PROGRAM AlarmsAndEventsCX7000
VAR
	events: ARRAY[0..7] OF ST_event;
	fbEvent_0: EventController;
	fbEvent_1: EventController;
	fbEvent_2: EventController;
	fbEvent_3: EventController;
	confirmAll: BOOL;
	clearAll: BOOL;
	resetAll: BOOL;
	initEvents : BOOL := FALSE;
	
END_VAR


IF NOT initEvents THEN
	initEvents := TRUE;
	
	// Info message
	events[0].severity := 0;
	events[0].needs_confirmation := FALSE;
	events[0].display_text := 'Nov izdelek na vhodnem traku.';
	events[0].cause_text := 'Prožena je fotocelica na vhodu';
	events[0].remedy_text := '';
	
	// Warning
	events[1].severity := 1;
	events[1].needs_confirmation := FALSE;
	events[1].display_text := 'Končan izdelek čaka na izhodu.';
	events[1].cause_text := 'Prožena je fotocelica na izhodu';
	events[1].remedy_text := 'Odstrani izdelek na izhodu.';
	
	// Error
	events[2].severity := 2;
	events[2].needs_confirmation := TRUE;
	events[2].display_text := 'Potiskač 1 v okvari.';
	events[2].cause_text := 'Aktivni sta obe končni stikali.';
	events[2].remedy_text := 'Preveri končna stikala, javi serviserju.';
	
	// Critical
	events[3].severity := 3;
	events[3].needs_confirmation := TRUE;
	events[3].display_text := 'Prekoračena omejitev iztega.';
	events[3].cause_text := 'Stevec korakov je vecji od dovoljene meje.';
	events[3].remedy_text := 'Prestavi v rocni nacin in referenciraj robota.';
	
END_IF

// Call the event controllers, each for an event
fbEvent_0(eventData := events[0]);
fbEvent_1(eventData := events[1]);
fbEvent_2(eventData := events[2]);
fbEvent_3(eventData := events[3]);

// Confirmation (if required)
fbEvent_2.confirm := confirmAll;
fbEvent_3.confirm := confirmAll;

// Clear
fbEvent_0.clear := clearAll;
fbEvent_1.clear := clearAll;
fbEvent_2.clear := clearAll;
fbEvent_3.clear := clearAll;

// Reset
fbEvent_0.reset := resetAll;
fbEvent_1.reset := resetAll;
fbEvent_2.reset := resetAll;
fbEvent_3.reset := resetAll;

END_PROGRAM
